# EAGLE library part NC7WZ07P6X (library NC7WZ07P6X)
Over-Voltage Tolerant Inputs Facilitate 5V to 3V Translation ; Ultra-Small MicroPak Packages; Proprietay Noise/EMI Reduction Circuitry ; Ultra-High Speed: tPZL 2.3ns (Typical) ; Power Down High Iimpedance Inputs/Outputs ; High IOL Output Drive: +24mA at 3V VCC ; Broad VCC Operating Range: 1.65V to 5.5V Source: Datasheet
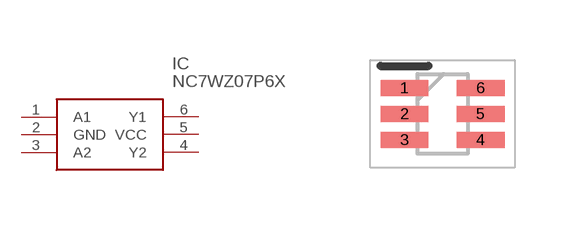
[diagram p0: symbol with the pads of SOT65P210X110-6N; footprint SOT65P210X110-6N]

Designator prefix IC

## NC7WZ07P6X (Arrow_Part_Number: NC7WZ07P6X; Arrow_Price-Stock: https://www.arrow.com/en/products/nc7wz07p6x/on-semiconductor?utm_currency=USD&region=europe; Description: Over-Voltage Tolerant Inputs Facilitate 5V to 3V Translation ; Ultra-Small MicroPak Packages; Proprietay Noise/EMI Reduction Circuitry ; Ultra-High Speed: tPZL 2.3ns (Typical) ; Power Down High Iimpedance Inputs/Outputs ; High IOL Output Drive: +24mA at 3V VCC ; Broad VCC Operating Range: 1.65V to 5.5V; Height: 1.1mm; Manufacturer_Name: onsemi; Manufacturer_Part_Number: NC7WZ07P6X; Mouser_Part_Number: 512-NC7WZ07P6X; Mouser_Price-Stock: https://www.mouser.co.uk/ProductDetail/onsemi-Fairchild/NC7WZ07P6X?qs=utFvTgNEmG4U5hUjGf3BdQ%3D%3D)  [SOT65P210X110-6N]
1  A1
2  GND
3  A2
4  Y2
5  VCC
6  Y1

## Footprint SOT65P210X110-6N (pad centres in mm)
NC7WZ07P6
smd 1.2 x 0.4: 1 -0.95,0.65; 2 -0.95,0; 3 -0.95,-0.65; 4 0.95,-0.65; 5 0.95,0; 6 0.95,0.65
